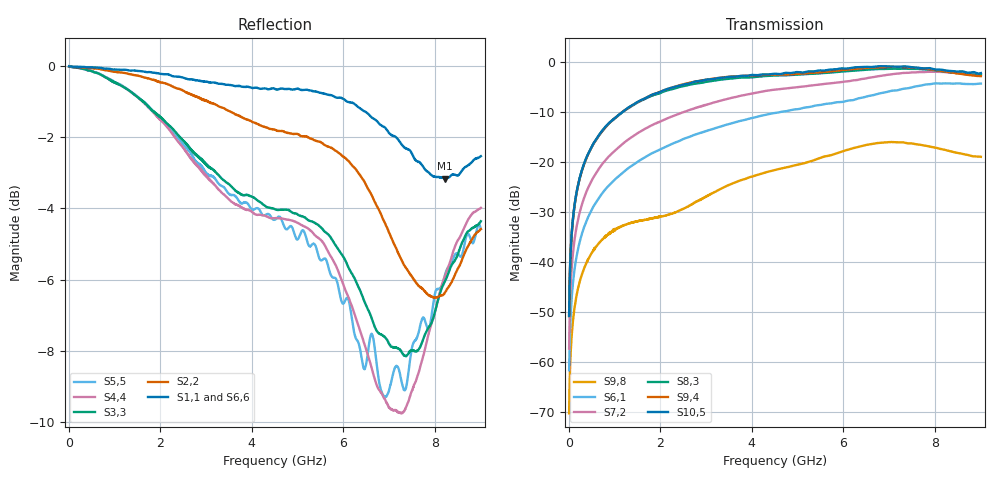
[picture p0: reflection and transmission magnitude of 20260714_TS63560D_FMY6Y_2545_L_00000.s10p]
# GHz S DB R 50
! CMT, SN0916, 25263762, 26.7.0
! Date: 15.07.2026 13:17:22
! Data: Format
! Freq S1.1:dB/Ang S1.2:dB/Ang S1.3:dB/Ang S1.4:dB/Ang S1.5:dB/Ang S1.6:dB/Ang S1.7:dB/Ang S1.8:dB/Ang S1.9:dB/Ang S1.10:dB/Ang
!  S2.1:dB/Ang S2.2:dB/Ang S2.3:dB/Ang S2.4:dB/Ang S2.5:dB/Ang S2.6:dB/Ang S2.7:dB/Ang S2.8:dB/Ang S2.9:dB/Ang S2.10:dB/Ang
!  S3.1:dB/Ang S3.2:dB/Ang S3.3:dB/Ang S3.4:dB/Ang S3.5:dB/Ang S3.6:dB/Ang S3.7:dB/Ang S3.8:dB/Ang S3.9:dB/Ang S3.10:dB/Ang
!  S4.1:dB/Ang S4.2:dB/Ang S4.3:dB/Ang S4.4:dB/Ang S4.5:dB/Ang S4.6:dB/Ang S4.7:dB/Ang S4.8:dB/Ang S4.9:dB/Ang S4.10:dB/Ang
!  S5.1:dB/Ang S5.2:dB/Ang S5.3:dB/Ang S5.4:dB/Ang S5.5:dB/Ang S5.6:dB/Ang S5.7:dB/Ang S5.8:dB/Ang S5.9:dB/Ang S5.10:dB/Ang
!  S6.1:dB/Ang S6.2:dB/Ang S6.3:dB/Ang S6.4:dB/Ang S6.5:dB/Ang S6.6:dB/Ang S6.7:dB/Ang S6.8:dB/Ang S6.9:dB/Ang S6.10:dB/Ang
!  S7.1:dB/Ang S7.2:dB/Ang S7.3:dB/Ang S7.4:dB/Ang S7.5:dB/Ang S7.6:dB/Ang S7.7:dB/Ang S7.8:dB/Ang S7.9:dB/Ang S7.10:dB/Ang
!  S8.1:dB/Ang S8.2:dB/Ang S8.3:dB/Ang S8.4:dB/Ang S8.5:dB/Ang S8.6:dB/Ang S8.7:dB/Ang S8.8:dB/Ang S8.9:dB/Ang S8.10:dB/Ang
!  S9.1:dB/Ang S9.2:dB/Ang S9.3:dB/Ang S9.4:dB/Ang S9.5:dB/Ang S9.6:dB/Ang S9.7:dB/Ang S9.8:dB/Ang S9.9:dB/Ang S9.10:dB/Ang
!  S10.1:dB/Ang S10.2:dB/Ang S10.3:dB/Ang S10.4:dB/Ang S10.5:dB/Ang S10.6:dB/Ang S10.7:dB/Ang S10.8:dB/Ang S10.9:dB/Ang S10.10:dB/Ang
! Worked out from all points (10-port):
!   2001 points, 10 MHz to 9 GHz, reference 50 ohm
!   strongest paths, dB at 10 MHz, 2.257 GHz, 4.505 GHz, 6.753 GHz, 9 GHz:
!     S10,5: -50.8, -5.1, -2.3, -0.8, -2.2
!     S9,4: -50.8, -5.1, -2.5, -1.0, -2.8
!     S8,3: -50.7, -5.4, -2.7, -1.4, -2.6
!     S7,2: -57.3, -10.9, -5.5, -2.8, -2.6
!     S6,1: -61.7, -16.4, -10.2, -6.4, -4.3
!     S9,8: -70.3, -30.3, -21.6, -16.2, -19.0
!   lowest |S11| = -3.2 dB at 8.209 GHz (marker M1), VSWR 5.56, Z = 11.1 - j23.5 ohm
!   |S11| at or under -10 dB: nowhere
